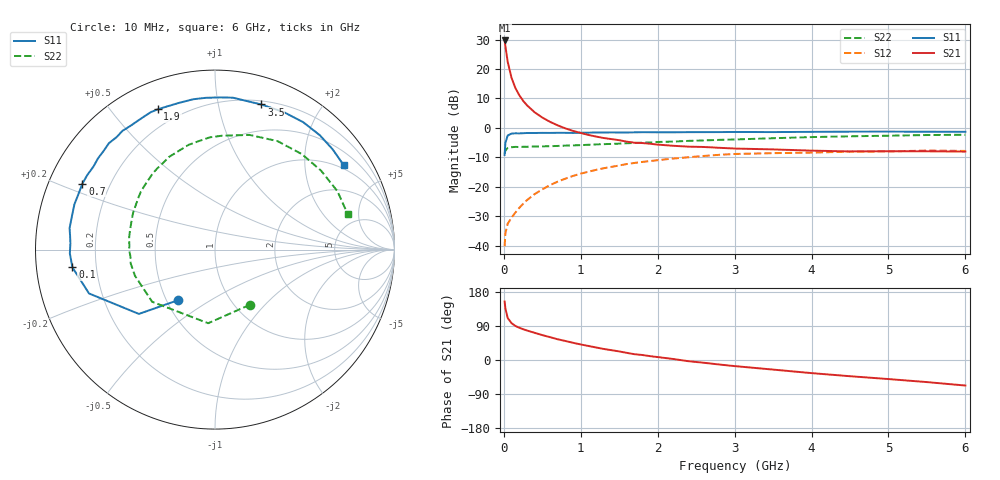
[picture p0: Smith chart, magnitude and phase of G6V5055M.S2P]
! SIEMENS Small Signal Semiconductors
! BFG193
! Si NPN RF Bipolar Junction Transistor in SOT223
! VCE = 0.5 V  IC = 55 mA
! Common Emitter S-Parameters:  August  1996
# GHz  S  MA  R  50
!  f  S11  S21  S12  S22
! GHz  MAG  ANG  MAG  ANG  MAG  ANG  MAG  ANG
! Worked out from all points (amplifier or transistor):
!   36 points, 10 MHz to 6 GHz, reference 50 ohm
!   highest |S21| = 29.7 dB at 10 MHz (marker M1)
!   |S21| within 3 dB of that: start of sweep to 26.27 MHz
!   unconditionally stable (mu >= 1): start of sweep to 16.02 MHz; 117.7 MHz to end of sweep
!   at 250 MHz: K = 1.27, MAG = 14.4 dB, |S12| = -25.8 dB
!   at 1.4 GHz: K = 1.25, MAG = 1.7 dB, |S12| = -13.2 dB
!   at 6 GHz: K = 1.08, MAG = -1.8 dB, |S12| = -7.8 dB
!   S11 on the Smith chart (normalised r, x): 10 MHz: 0.58, -0.37; 100 MHz: 0.11, -0.06; 700 MHz: 0.10, +0.23; 1.9 GHz: 0.12, +0.67; 3.5 GHz: 0.23, +1.34; 6 GHz: 0.87, +3.11
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0.01  0.3469 -125.9  30.54 154.4  0.0098 61.9  0.3636 -57.7
0.02  0.5552 -139.8  24.6 136.4  0.0162 52.9  0.412 -95.3
0.05  0.7432 -160.8  13.26 110.8  0.0236 41.4  0.4551 -140.3
0.1  0.8006 -172.9  7.074 97.2  0.0299 45.3  0.4692 -162.0
0.15  0.809 -178.5  4.755 89.9  0.0365 50.5  0.4759 -170.6
0.2  0.8064 177.5  3.604 85.2  0.0437 54.6  0.4729 -175.6
0.25  0.8116 174.3  2.893 81.3  0.0513 57.0  0.4782 -179.8
0.3  0.819 171.6  2.425 77.9  0.0592 58.8  0.4776 177.5
0.4  0.8187 166.5  1.842 71.7  0.0749 59.8  0.4829 172.0
0.5  0.823 162.1  1.499 65.7  0.0905 59.0  0.4854 167.4
0.6  0.8212 157.9  1.267 60.3  0.1068 57.9  0.4885 163.5
0.7  0.8251 153.5  1.104 54.7  0.1222 56.2  0.4937 159.8
0.9  0.82 145.7  0.888 45.4  0.1528 51.7  0.5043 152.0
1.1  0.8291 138.5  0.759 37.0  0.1803 47.1  0.5165 145.5
1.6  0.8363 121.4  0.583 18.8  0.2434 33.6  0.5489 129.0
1.9  0.8443 112.2  0.538 10.2  0.2734 25.8  0.5663 119.6
2.2  0.8416 104.0  0.497 2.7  0.3015 17.3  0.5855 110.3
2.8  0.8485 88.0  0.459 -11.9  0.349 1.8  0.6261 92.7
3.5  0.8486 72.3  0.431 -25.3  0.3724 -16.5  0.6674 73.2
4.5  0.8634 55.3  0.398 -42.8  0.3949 -35.0  0.7193 47.6
5.5  0.8613 40.5  0.4 -58.3  0.4124 -55.8  0.7559 25.4
6  0.8576 33.4  0.396 -67.4  0.4064 -67.6  0.7649 15.0
